PROGRAM MAIN

VAR CONSTANT
    cInitSource			: ST_MA_MultiArray_InitPars 
							:= ( eTypeCode := eMA_TypeCode_LCOMPLEX, nDims := 1, aDimSizes := [cBufferLength]);	
END_VAR

VAR
	(* Input *)
	nInputSelection		: UDINT := 1;				// Switch between hardware and function generator	
	nSample				: UDINT;                            
	
	(* Signal Generator *)
	fbFunctionGenerator_re	: FB_FunctionGenerator; // real part signal generator
	fSetFrequency_re		: LREAL := 200;			// Hz
	fSetAmplitude_re		: LREAL := 13;			// peak amplitude of sin signal		
	fbFunctionGenerator_im	: FB_FunctionGenerator; // imaginary part signal generator
	fSetFrequency_im		: LREAL := 600;			// Hz
	fSetAmplitude_im		: LREAL := 7;			// peak amplitude of sin signal		
    aBuffer_re			: ARRAY[1..cOversamples] OF LREAL;                    
	aBuffer_im			: ARRAY[1..cOversamples] OF LREAL;
	
	(* Source buffers *)		
	aBuffer			    : ARRAY[1..cOversamples] OF LCOMPLEX;			
	fbSource			: FB_CMA_Source :=(	stInitPars := cInitSource, 
											nOwnID := eID_Source, 
											aDestIDs := [eID_FFT]);		// Initialize source buffers
	(* Result buffers *)										
	aSpectrumResult		: ARRAY[1..cFFTResult] OF LCOMPLEX;				// local result variable <- from sink
    fbSink				: FB_CMA_Sink := (nOwnID := eID_Sink);			// Initialize sink buffers
	
	
	(* post-processing of fft *)
	nCountResults		: ULINT;            				// increments for every fft calculation
	bCalculate			: BOOL;             				// true if fft calculation ready	
	SpectrumAbs         : ARRAY[1..cFFTResult] OF LREAL; 	// magnitude spectrum variable 
	(* max amplitude calculation *)
	fMaxAmpl			: LREAL;
	nIdxOfMaxAmpl		: UDINT;		// index of max amplitude in spectrum result array 
	(* frequency calculation *)
	fSampleTaskCycleTime: LREAL := 1; 	// ms
	fSampleRate			: LREAL;		// Hz  ( sample rate = oversampling factor / cycle time )
	fResolution			: LREAL;		// Hz/Idx
	fFrequency			: LREAL;		// Hz	
	
	(* error monitoring *)
	fbErrHist			: FB_HRErrHist;

END_VAR

(* Input *) 

(* signal generator *)		
// generate real part of signal
fbFunctionGenerator_re(	fFrequency 	:= fSetFrequency_re,
						fAmplitude 	:= fSetAmplitude_re,
						eFunction 	:= E_FunctionType.Sine,
						aSignal		:= aBuffer_re);
// generate imaginary part of signal		
fbFunctionGenerator_im(	fFrequency 	:= fSetFrequency_im,
						fAmplitude 	:= fSetAmplitude_im,
						eFunction 	:= E_FunctionType.Sine,
						aSignal		:= aBuffer_im);
// combine to complex signal
FOR nSample := 1 TO cOversamples DO
	aBuffer[nSample].re := aBuffer_re[nSample];
	aBuffer[nSample].im := aBuffer_im[nSample];			
END_FOR        							
					

(* Call source to collect data *)
fbSource.Input1DStd(pDataIn 		:= ADR(aBuffer),
					nDataInSize 	:= SIZEOF(aBuffer), 
					eElementType 	:= eMA_TypeCode_LCOMPLEX,
					nOptionPars		:= cCMA_Option_MarkInterruption ); 
IF fbSource.bError THEN
	fbErrHist.AddError(bErr:=TRUE, hrErrCode:=fbSource.hrErrorCode, sErrSource:='MAIN.fbSource'); // error monitoring
	// ToDo: if error
END_IF


(* Push results to sink *)
fbSink.Output1DStd(	pDataOut 		:= ADR(aSpectrumResult), 
					nDataOutSize 	:= SIZEOF(aSpectrumResult), 
					eElementType 	:= eMA_TypeCode_LCOMPLEX, 
					nOptionPars		:= 0,
					bNewResult		=> bCalculate );
IF fbSink.bError THEN
	fbErrHist.AddError(bErr:=TRUE, hrErrCode:=fbSink.hrErrorCode, sErrSource:='MAIN.fbSink'); // error monitoring
	// ToDo: if error
END_IF

(* post-process fft result *)
IF bCalculate THEN
	nCountResults := fbSink.nCntResults;
	
	// Calculate absolute value as aSpectrumResult is of complex type
	FOR nSample := 1 TO cFFTResult DO			   	   
	   SpectrumAbs[nSample] := SQRT(aSpectrumResult[nSample].re * aSpectrumResult[nSample].re + aSpectrumResult[nSample].im * aSpectrumResult[nSample].im);
       
	   // scale spectrum
	   IF nSample = 1 THEN
		   SpectrumAbs[nSample] := SpectrumAbs[nSample]/cFFTLength;   // scale DC value
	   ELSE
		   SpectrumAbs[nSample] := 2*SpectrumAbs[nSample]/cFFTLength; // scale frequencies not equal to 0
	   END_IF
	   
	END_FOR;
	
	IF NOT LrealIsNaN(SpectrumAbs[1]) THEN
		
		// Calculate max amplitude in spectrum
		fMaxAmpl := 0;
		FOR nSample:=1 TO cFFTResult/2+1 DO
			IF SpectrumAbs[nSample] > fMaxAmpl THEN
				fMaxAmpl := SpectrumAbs[nSample];
				nIdxOfMaxAmpl := nSample;
			END_IF
		END_FOR
		
		// Calculate frequency for max amplitude [ frequency = index * (sample rate / FFT length) ]
		fSampleRate := cOversamples * (1000.0 / fSampleTaskCycleTime);
		fResolution := fSampleRate / cFFTLength;
		fFrequency := (nIdxOfMaxAmpl-1) * fResolution;	 // -1 to consider DC = 0*fResolution
	END_IF
	// ToDo: if new result is ready
	
END_IF

END_PROGRAM
